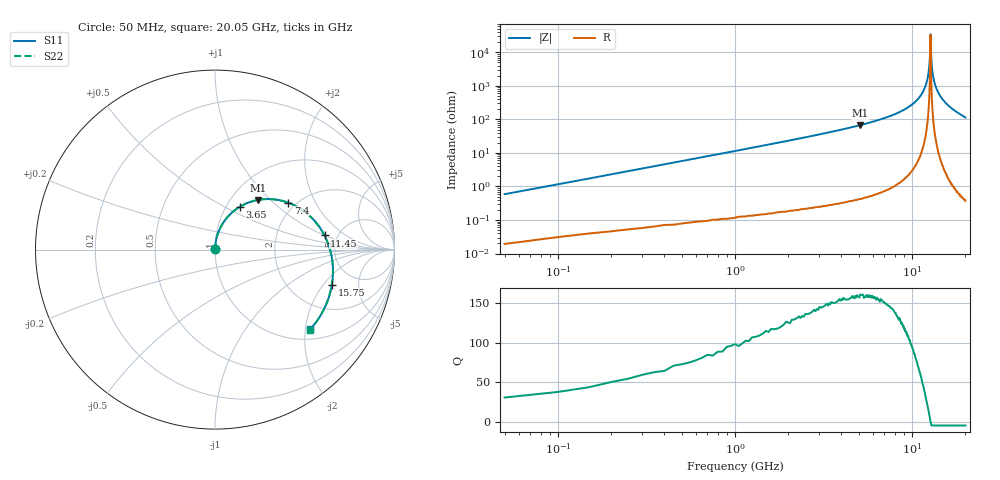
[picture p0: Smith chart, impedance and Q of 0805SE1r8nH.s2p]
! AVX Thin Film Operation		Date: May 2002
! Description: Accu-L® Series, Thin Film, SMD, RF Inductors
! Part Number: L08051R8CEWTR
! 50 MHz  -  20.05 GHz
! Serial Measurements
# mhz S db R 50
!	S11		S21		S12		S22
!	dB	Phase	dB	Phase	dB	Phase	dB	Phase
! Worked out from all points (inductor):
!   401 points, 50 MHz to 20.05 GHz, reference 50 ohm
!   read as 1/Y11, port 2 shorted: L = 1.83 nH near 150 MHz
!   highest Q = 161 at 5.1 GHz (marker M1), where L = 2.1 nH
!   self-resonance near 12.7 GHz
!   S11 on the Smith chart (normalised r, x): 50 MHz: 1.00, +0.01; 3.65 GHz: 1.16, +0.60; 7.4 GHz: 1.82, +1.25; 11.45 GHz: 3.93, +1.00; 15.75 GHz: 3.37, -2.44; 20.05 GHz: 1.25, -2.13
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50  -47.39 87.2  -0.00 -0.4  -0.00 -0.4  -47.39 87.2
100  -41.58 87.0  -0.00 -0.8  -0.00 -0.8  -41.58 87.0
200  -35.67 86.7  -0.01 -1.7  -0.01 -1.7  -35.67 86.7
250  -33.76 86.4  -0.01 -2.1  -0.01 -2.1  -33.76 86.4
350  -30.88 85.8  -0.01 -2.9  -0.01 -2.9  -30.88 85.8
450  -28.73 85.1  -0.01 -3.8  -0.01 -3.8  -28.73 85.1
600  -26.26 84.0  -0.02 -5.0  -0.02 -5.0  -26.26 84.0
900  -22.79 81.6  -0.03 -7.5  -0.03 -7.5  -22.79 81.6
1350  -19.33 78.1  -0.06 -11.2  -0.06 -11.2  -19.33 78.0
1900  -16.45 73.7  -0.11 -15.7  -0.11 -15.7  -16.45 73.6
2600  -13.86 68.1  -0.20 -21.4  -0.20 -21.4  -13.86 68.0
3400  -11.71 61.8  -0.32 -27.7  -0.32 -27.7  -11.71 61.7
3650  -11.16 59.9  -0.37 -29.7  -0.37 -29.7  -11.16 59.8
5100  -8.69 48.9  -0.66 -40.7  -0.66 -40.7  -8.69 48.8
6750  -6.84 37.1  -1.04 -52.5  -1.04 -52.5  -6.84 37.0
7400  -6.29 32.7  -1.19 -57.0  -1.19 -57.0  -6.29 32.6
10050  -4.74 15.7  -1.81 -74.1  -1.81 -74.1  -4.74 15.6
11450  -4.21 7.3  -2.10 -82.5  -2.10 -82.5  -4.21 7.2
13400  -3.71 -3.8  -2.44 -93.7  -2.44 -93.7  -3.71 -4.0
15750  -3.35 -16.7  -2.73 -106.6  -2.73 -106.6  -3.35 -16.9
16750  -3.26 -22.1  -2.81 -112.0  -2.81 -112.0  -3.26 -22.3
20050  -3.19 -39.8  -2.87 -129.8  -2.87 -129.8  -3.20 -40.0
